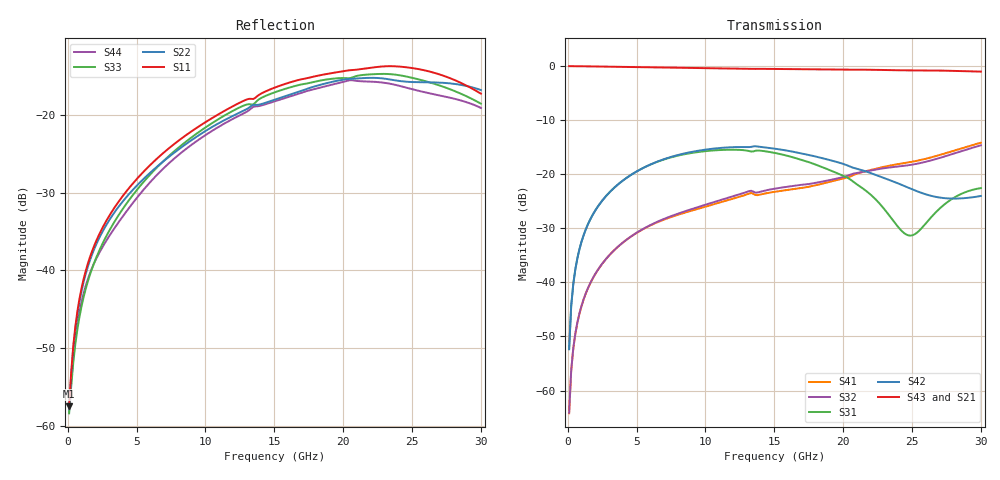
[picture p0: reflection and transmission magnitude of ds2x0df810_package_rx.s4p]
# GHz S DB R 50
! S-Parameters data
! Freq  dbS11  angS11  dbS12  angS12  dbS13  angS13  dbS14  angS14
!  dbS21  angS21  dbS22  angS22  dbS23  angS23  dbS24  angS24
!  dbS31  angS31  dbS32  angS32  dbS33  angS33  dbS34  angS34
!  dbS41  angS41  dbS42  angS42  dbS43  angS43  dbS44  angS44
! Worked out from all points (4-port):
!   200 points, 100 MHz to 30 GHz, reference 50 ohm
!   strongest paths, dB at 100 MHz, 7.613 GHz, 15.13 GHz, 22.64 GHz, 30 GHz:
!     S43: 0.0, -0.3, -0.5, -0.7, -1.0
!     S21: 0.0, -0.3, -0.6, -0.7, -1.1
!     S42: -52.4, -16.7, -15.3, -20.4, -24.0
!     S31: -52.3, -16.8, -16.1, -25.4, -22.6
!     S32: -64.1, -27.6, -22.6, -19.0, -14.7
!     S41: -64.2, -27.8, -23.2, -18.8, -14.2
!   lowest |S11| = -57.5 dB at 100 MHz (marker M1), VSWR 1.00, Z = 50.1 + j0.0735 ohm
!   |S11| at or under -10 dB: start of sweep to end of sweep
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0.1  -57.46 33.2  -0.01 -0.9  -52.34 84.9  -64.22 -101.0
     -0.01 -0.9  -57.74 34.2  -64.13 -101.9  -52.36 84.9
     -52.34 84.9  -64.13 -101.9  -58.36 26.7  -0.01 -0.8
     -64.22 -101.0  -52.36 84.9  -0.01 -0.8  -58.16 30.6
0.5507538  -47.21 65.4  -0.02 -4.8  -37.58 83.9  -49.54 -97.2
           -0.02 -4.8  -47.56 72.4  -49.48 -97.9  -37.60 84.0
           -37.58 83.9  -49.48 -97.9  -49.49 61.1  -0.02 -4.6
           -49.54 -97.2  -37.60 84.0  -0.02 -4.6  -48.75 69.1
1.602513  -38.34 56.6  -0.05 -13.8  -28.51 74.6  -40.35 -106.2
          -0.05 -13.8  -38.75 77.2  -40.31 -107.7  -28.53 75.0
          -28.51 74.6  -40.31 -107.7  -40.60 54.0  -0.05 -13.2
          -40.35 -106.2  -28.53 75.0  -0.05 -13.2  -40.40 74.3
6.711055  -25.25 -10.8  -0.25 -56.3  -17.51 32.9  -28.67 -152.7
          -0.25 -56.3  -26.31 66.7  -28.56 -157.4  -17.46 34.6
          -17.51 32.9  -28.56 -157.4  -26.34 -11.8  -0.24 -53.8
          -28.67 -152.7  -17.46 34.6  -0.24 -53.8  -27.30 71.9
19.78291  -14.45 -146.9  -0.65 -164.0  -20.05 -64.1  -20.92 113.7
          -0.65 -164.0  -15.54 -3.4  -20.66 93.6  -17.91 -79.0
          -20.05 -64.1  -20.66 93.6  -15.27 -128.4  -0.62 -156.4
          -20.92 113.7  -17.91 -79.0  -0.62 -156.4  -15.87 -8.4
24.89146  -13.95 165.3  -0.86 152.7  -31.35 -40.4  -17.74 73.1
          -0.86 152.7  -15.77 -38.4  -18.27 50.3  -22.66 -159.6
          -31.35 -40.4  -18.27 50.3  -15.19 -167.8  -0.78 162.9
          -17.74 73.1  -22.66 -159.6  -0.78 162.9  -16.64 -49.5
30  -17.27 124.7  -1.13 106.6  -22.56 -31.5  -14.17 28.1
    -1.13 106.6  -16.81 -75.0  -14.65 5.8  -24.02 111.3
    -22.56 -31.5  -14.65 5.8  -18.56 162.0  -1.02 119.3
    -14.17 28.1  -24.02 111.3  -1.02 119.3  -19.11 -82.6
